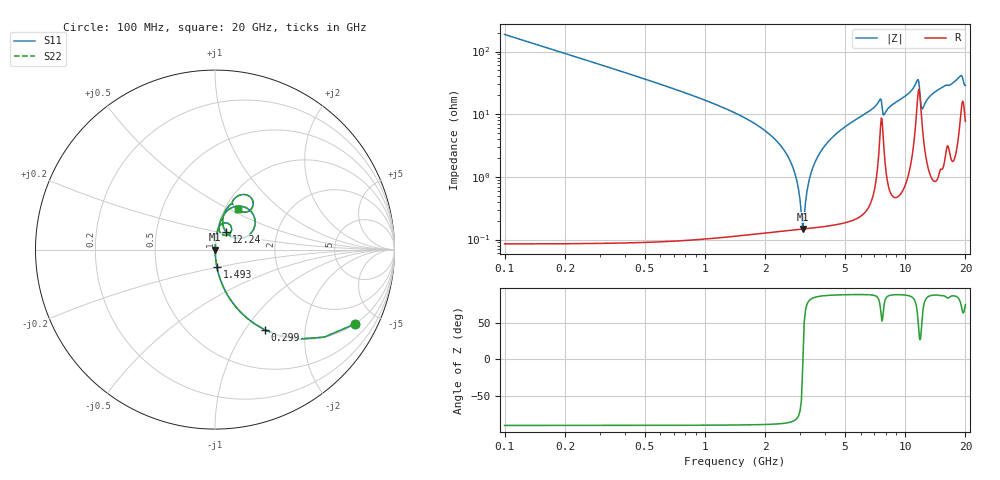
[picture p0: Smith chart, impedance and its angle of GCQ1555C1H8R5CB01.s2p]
!Murata Part Number: GCQ1555C1H8R5CB01
!These Parameters are Measured in Series Mode Connection
!Data Generated on Mar 13, 2026
!  o--ll--o
!Port1  Port2
!  o------o
!Operation Temp=25[degC], DC Bias Voltage=0[V]
!Freq. Start=100[MHz] Stop=20[GHz] 401[Steps]
# Hz S RI R 50
!Freq.(Hz) S11(Real) S11(Imag) S21(Real) S21(Imag) S12(Real) S12(Imag) S22(Real) S22(Imag)
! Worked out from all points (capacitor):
!   401 points, 100 MHz to 20 GHz, reference 50 ohm
!   read as one part in series: C = 8.5 pF near 199.5 MHz
!   lowest |Z| = 147 mohm at 3.085 GHz (marker M1)
!   series resonance near 3.088 GHz, so ESL is about 310 pH
!   S11 on the Smith chart (normalised r, x): 100 MHz: 1.00, -3.74; 299 MHz: 1.00, -1.24; 1.493 GHz: 1.00, -0.19; 12.24 GHz: 1.11, +0.22; 20 GHz: 1.15, +0.55
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1e8  0.7776 -0.4156  0.2224 0.4156  0.2224 0.4156  0.7776 -0.4156
2.99e8  0.2782 -0.4474  0.7218 0.4474  0.7218 0.4474  0.2782 -0.4474
6.4725e8  0.0718 -0.2564  0.9282 0.2564  0.9282 0.2564  0.0718 -0.2564
1.493e9  0.0103 -0.095  0.9897 0.095  0.9897 0.095  0.0103 -0.095
2.5875e9  0.00185 -0.0216  0.9982 0.0216  0.9982 0.0216  0.00185 -0.0216
2.83625e9  0.00153 -0.0104  0.9985 0.0104  0.9985 0.0104  0.00153 -0.0104
2.9855e9  0.00147 -0.00412  0.9985 0.00412  0.9985 0.00412  0.00147 -0.00412
3.085e9  0.00147 -0.000135  0.9985 0.000135  0.9985 0.000135  0.00147 -0.000135
3.43325e9  0.00169 0.0129  0.9983 -0.0129  0.9983 -0.0129  0.00169 0.0129
3.83125e9  0.0023 0.0266  0.9977 -0.0266  0.9977 -0.0266  0.0023 0.0266
4.42825e9  0.00376 0.0453  0.9962 -0.0453  0.9962 -0.0453  0.00376 0.0453
6.7665e9  0.0175 0.1151  0.9825 -0.1151  0.9825 -0.1151  0.0175 0.1151
7.51275e9  0.0737 0.1458  0.9263 -0.1458  0.9263 -0.1458  0.0737 0.1458
7.861e9  0.0329 0.0899  0.9671 -0.0899  0.9671 -0.0899  0.0329 0.0899
1.005e10  0.0438 0.1861  0.9562 -0.1861  0.9562 -0.1861  0.0438 0.1861
1.15425e10  0.204 0.2089  0.796 -0.2089  0.796 -0.2089  0.204 0.2089
1.204e10  0.0976 0.0695  0.9024 -0.0695  0.9024 -0.0695  0.0976 0.0695
1.2239e10  0.0616 0.0982  0.9384 -0.0982  0.9384 -0.0982  0.0616 0.0982
1.338325e10  0.0466 0.1859  0.9534 -0.1859  0.9534 -0.1859  0.0466 0.1859
1.67165e10  0.0958 0.2568  0.9042 -0.2568  0.9042 -0.2568  0.0958 0.2568
1.89055e10  0.1912 0.2972  0.8088 -0.2972  0.8088 -0.2972  0.1912 0.2972
2e10  0.1292 0.2243  0.8708 -0.2243  0.8708 -0.2243  0.1292 0.2243
